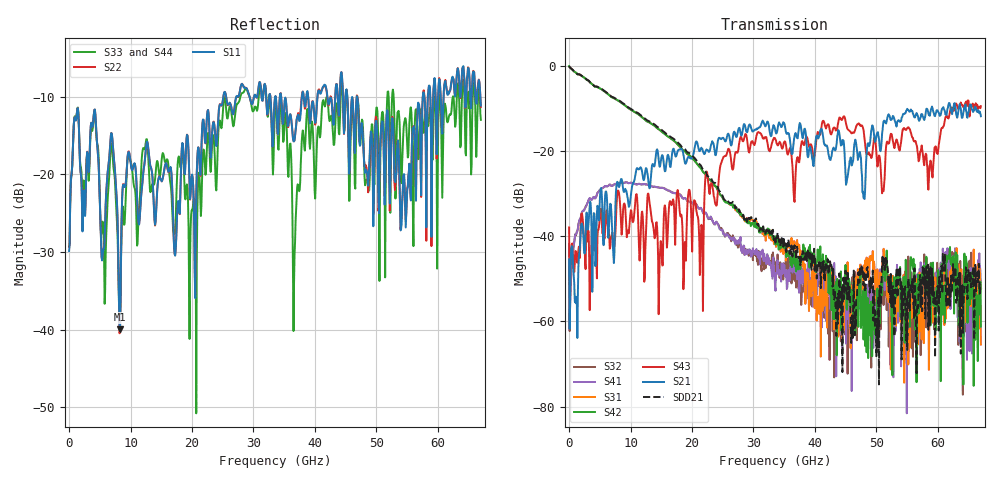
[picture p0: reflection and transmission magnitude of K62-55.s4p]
!Agilent Technologies,N5247A,US50470101,A.10.25.02
!Agilent N5247A: A.10.25.02
!Date: Tuesday, May 12, 2015 13:43:30
!Correction: Sdd11(Full 4 Port(1,2,3,4))
!Sdc11(Full 4 Port(1,2,3,4))
!Sdd12(Full 4 Port(1,2,3,4))
!Sdc12(Full 4 Port(1,2,3,4))
!Scd11(Full 4 Port(1,2,3,4))
!Scc11(Full 4 Port(1,2,3,4))
!Scd12(Full 4 Port(1,2,3,4))
!Scc12(Full 4 Port(1,2,3,4))
!Sdd21(Full 4 Port(1,2,3,4))
!Sdc21(Full 4 Port(1,2,3,4))
!Sdd22(Full 4 Port(1,2,3,4))
!Sdc22(Full 4 Port(1,2,3,4))
!Scd21(Full 4 Port(1,2,3,4))
!Scc21(Full 4 Port(1,2,3,4))
!Scd22(Full 4 Port(1,2,3,4))
!Scc22(Full 4 Port(1,2,3,4))
!Balanced Topology: BBAL
!S4P File: Measurements: <Sdd11,Sdc11,Sdd12,Sdc12>,
!<Scd11,Scc11,Scd12,Scc12>,
!<Sdd21,Sdc21,Sdd22,Sdc22>,
!<Scd21,Scc21,Scd22,Scc22>:
# Hz S  dB  R 50
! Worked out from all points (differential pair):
!   801 points, 10 MHz to 67 GHz, reference 50 ohm
!   strongest paths, dB at 10 MHz, 16.76 GHz, 33.51 GHz, 50.25 GHz, 67 GHz:
!     S21: -45.4, -20.7, -14.8, -15.5, -11.8
!     S43: -37.9, -32.2, -17.0, -23.0, -9.5
!     S42: -0.1, -17.2, -40.8, -57.4, -61.2
!     S31: -0.1, -17.3, -40.7, -52.4, -65.4
!     S41: -41.7, -29.8, -51.5, -55.0, -50.6
!     S32: -47.6, -29.6, -46.3, -65.5, -52.2
!   taken as a pair (ports 2,1 in; 4,3 out), SDD21 dB: 0.0, -16.9, -40.5, -66.1, -51.3
!   lowest |S11| = -39.9 dB at 8.216 GHz (marker M1), VSWR 1.02, Z = 49.1 - j0.505 ohm
!   |S11| at or under -10 dB: start of sweep to 25.1 GHz; 34.5 GHz to 37.88 GHz (3.386 GHz wide, 9.36 % of centre); 46.88 GHz to 57.55 GHz (10.68 GHz wide, 20.5 % of centre)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
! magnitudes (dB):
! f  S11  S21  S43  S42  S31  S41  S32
! 10 MHz  -29.9  -45.4  -37.9  -0.1  -0.1  -41.7  -47.6
! 4.029 GHz  -12.3  -34.6  -43.4  -4.7  -4.7  -30.8  -30.8
! 8.216 GHz  -39.9  -28.1  -31.0  -8.4  -8.3  -27.5  -27.5
! 21.53 GHz  -16.7  -19.2  -37.3  -24.2  -24.2  -33.5  -33.6
! 28.06 GHz  -8.4  -16.4  -16.9  -34.8  -35.3  -42.3  -42.7
! 46.23 GHz  -11.8  -22.1  -15.7  -61.9  -55.4  -51.3  -58.9
! 67 GHz  -11.1  -11.8  -9.5  -61.2  -65.4  -50.6  -52.2
